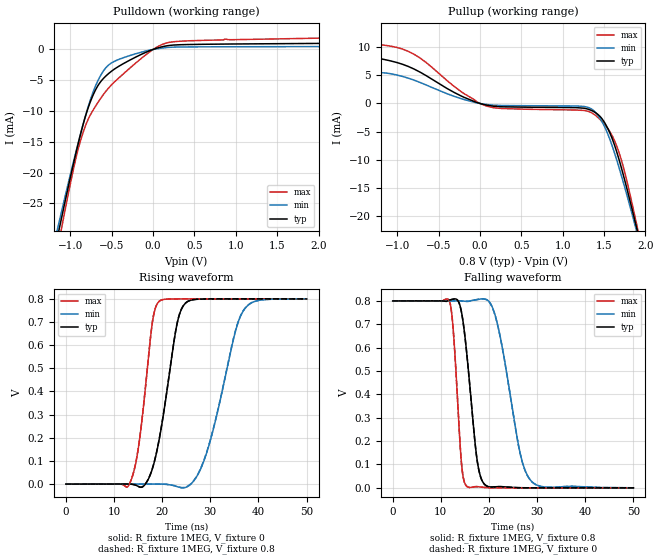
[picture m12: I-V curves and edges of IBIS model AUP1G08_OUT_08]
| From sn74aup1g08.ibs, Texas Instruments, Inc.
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[Model]   AUP1G08_OUT_08
Model_type  Output
Vref =   0
Rref =   1E6
Cref =   30p
Vmeas =   0.4
| variable   typ   min   max
C_comp   2.77pF   2.26pF   3.38pF
| C_pullup   2.83pF   2.27pF   3.38pF
| C_pulldown   2.71pF   2.26pF   3.15pF
[Temperature Range]   40   100   -40
| Ambient temperature   25   85   -40
[Voltage range]   0.8   0.8   0.8
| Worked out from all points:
|   slope of the pulldown table from 0 to 0.12 V, typ, clamps not added: 257 ohm
|   slope of the pullup table from 0 to 0.12 V, typ, clamps not added: 309 ohm
|   rising waveform, R_fixture 1MEG, V_fixture 0: 20-80 % time 3.57ns typ, 5.37ns min, 2.54ns max; typ from 0 V to 0.8 V
|   falling waveform, R_fixture 1MEG, V_fixture 0.8: 20-80 % time 2.23ns typ, 3.95ns min, 1.38ns max; typ from 0.8 V to 0 V
|   rising waveform, R_fixture 1MEG, V_fixture 0.8: 20-80 % time 3.57ns typ, 5.37ns min, 2.54ns max; typ from 0 V to 0.8 V
|   falling waveform, R_fixture 1MEG, V_fixture 0: 20-80 % time 2.23ns typ, 3.95ns min, 1.38ns max; typ from 0.8 V to 0 V
[Pulldown]
| AUP1G08_OUT_08
|   Voltage   I(typ)   I(min)   I(max)
-3.6V     -200.4mA   -184.8mA   -219.2mA
-1.155V   -30.45mA   -29.14mA   -32.46mA
-1.105V   -27.28mA   -26.24mA   -28.94mA
-940mV    -17.25mA   -17.03mA   -18.09mA
-865mV    -13.14mA   -13.11mA   -14.28mA
-745mV    -8.046mA   -7.664mA   -10.32mA
-630mV    -5.174mA   -4.131mA   -7.88mA
-470mV    -3.218mA   -1.946mA   -5.328mA
5mV       23.8uA     12.51uA    45.54uA
210mV     667.8uA    349.8uA    1.181mA
875mV     872.7uA    431.9uA    1.671mA
7.2V      1.459mA    578.6uA    3.138mA
[Pullup]
| AUP1G08_OUT_08
|   Voltage   I(typ)   I(min)   I(max)
-3.6V     2.784mA    339.3uA    9.474mA
-2.56V    3.921mA    664.1uA    11.14mA
-2.01V    6.261mA    1.27mA     13.38mA
-1.185V   7.904mA    5.467mA    10.42mA
-800mV    6.148mA    4.167mA    8.778mA
80mV      -287uA     -177.3uA   -461.9uA
1.285V    -921uA     -607.2uA   -1.305mA
1.455V    -2.356mA   -2.739mA   -2.902mA
1.625V    -7.338mA   -8.734mA   -6.561mA
1.74V     -13.1mA    -14.39mA   -11.68mA
1.905V    -22.8mA    -23.34mA   -22.24mA
7.2V      -397.1mA   -367.6mA   -431.9mA
[Ramp]
| AUP1G08_OUT_08
| variable   typ   min   max
dV/dt_r   0.49/3.66E-09   0.49/5.51E-09   0.49/2.60E-09
dV/dt_f   0.48/2.26E-09   0.48/4.00E-09   0.48/1.40E-09
R_load = 1MEG
[Rising Waveform]
| AUP1G08_OUT_08
R_fixture =   1MEG
C_fixture =   0
L_fixture =   0
V_fixture =   0
V_fixture_min = 0
V_fixture_max = 0
|   Time   V(typ)   V(min)   V(max)
0s        31.72nV    235.4nV    1.152nV
13.18ns   73.62uV    -83.35uV   -438.3uV
16.72ns   6.265mV    318.1uV    455.2mV
18.12ns   76.08mV    285.5uV    716.5mV
19.46ns   201.4mV    136uV      790.4mV
22.98ns   679.2mV    -9.969mV   799.7mV
24.87ns   781.5mV    -14.23mV   799.8mV
29.17ns   799.4mV    129.8mV    799.9mV
36.9ns    799.8mV    749mV      799.9mV
50ns      799.8mV    799.6mV    799.9mV
[Falling Waveform]
| AUP1G08_OUT_08
R_fixture =   1MEG
C_fixture =   0
L_fixture =   0
V_fixture =   0.8
V_fixture_min = 0.8
V_fixture_max = 0.8
|   Time   V(typ)   V(min)   V(max)
0s        800mV      800mV      800mV
11.77ns   803.2mV    800mV      799.6mV
12.63ns   807.8mV    800.1mV    660mV
14.3ns    749.6mV    799.6mV    100.3mV
15.42ns   567mV      798mV      6.096mV
17.51ns   122.2mV    805.7mV    5.178mV
19.24ns   11.85mV    807.6mV    1.354mV
21.66ns   5.077mV    709.1mV    152.6uV
28.57ns   277.9uV    34.25mV    87.41uV
50ns      166.9uV    375.4uV    86.96uV
[Rising Waveform]
| AUP1G08_OUT_08
R_fixture =   1MEG
C_fixture =   0
L_fixture =   0
V_fixture =   0.8
V_fixture_min = 0.8
V_fixture_max = 0.8
|   Time   V(typ)   V(min)   V(max)
0s        166.8uV    317.6uV    87.04uV
13.18ns   235.1uV    234.5uV    -192.3uV
16.71ns   6.776mV    628.7uV    454.5mV
18.11ns   76.95mV    592.4uV    716.8mV
19.46ns   202.4mV    439.6uV    790.6mV
22.97ns   679.7mV    -9.356mV   799.8mV
24.85ns   781.7mV    -13.22mV   799.9mV
29.15ns   799.6mV    130.8mV    800mV
36.86ns   800mV      749.5mV    800mV
50ns      800mV      799.9mV    800mV
[Falling Waveform]
| AUP1G08_OUT_08
R_fixture =   1MEG
C_fixture =   0
L_fixture =   0
V_fixture =   0
V_fixture_min = 0
V_fixture_max = 0
|   Time   V(typ)   V(min)   V(max)
0s        799.8mV    799.7mV    799.9mV
11.77ns   803mV      799.7mV    799.2mV
12.63ns   807.4mV    799.8mV    659.3mV
14.3ns    748.8mV    799.3mV    99.77mV
15.42ns   565.9mV    797.7mV    5.962mV
17.51ns   122mV      805.3mV    5.09mV
19.23ns   11.67mV    806.7mV    1.269mV
21.65ns   4.902mV    708.3mV    66.07uV
28.55ns   110.6uV    33.92mV    377.6nV
50ns      -88.12nV   54.98uV    -78.72nV
